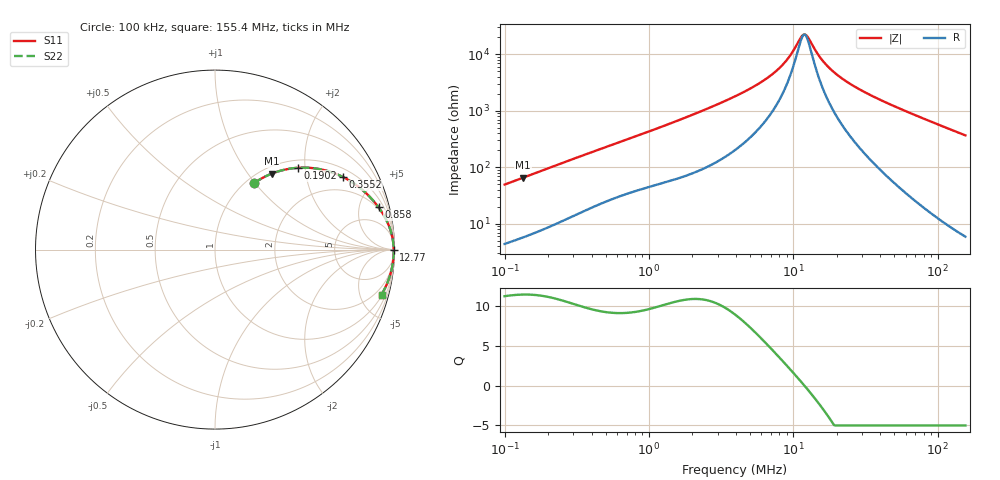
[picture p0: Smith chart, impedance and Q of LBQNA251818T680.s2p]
! LBQNA251818T680  S-PARAMETER MODEL  ( General Type )
! Model Generated by TAIYO YUDEN Corporation (http://www.ty-top.com)
! Version 1.0
! TAIYO YUDEN Control No. 191025NI43SB-FBB
! Copyright(c) 2019 TAIYO YUDEN CO.,LTD. All Rights Reserved.
! Product Description (link to TY-COMPAS)
! https://ds.yuden.co.jp/TYCOMPAS/or/detail?pn=LBQNA251818T680K&u=M
! Products Name : Inductors
! Characteristics :
!  Inductance : 68 uH , SRF(min) : 9.5 MHz , DC Resistance(max) : 1.95 Ohm
!  Rated Current : Saturation :70 mA , Temp Rise : 210 mA (20 degC)
!  Case Size : 2.5 x 1.8 / 0.098 x 0.071 [mm/inch] , Thickness : 1.8 / 0.071 [mm/inch]
!  (Conditions: Temperature = 25 degC , DC Bias Current/Voltage = 0A / 0V)
! External Node Assignments :
!  1  o---GGG---o  2
! GND o---------o GND
! Frequency Range : 0.1MHz  -  155.401204MHz  [ 402 STEP ]
# MHz S RI R 50
! Freq[MHz].  S11 Real  S11 Imag  S21 Real  S21 Imag  S12 Real  S12 Imag  S22 Real  S22 Imag
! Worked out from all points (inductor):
!   401 points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, 100 kHz to 155.4 MHz, reference 50 ohm
!   read as one part in series: L = 77.7 uH near 103.7 kHz
!   highest Q = 11.4 at 134.2 kHz (marker M1), where L = 77.6 uH
!   self-resonance near 11.87 MHz
!   S11 on the Smith chart (normalised r, x): 100 kHz: 1.09, +0.99; 190.2 kHz: 1.16, +1.83; 355.2 kHz: 1.34, +3.30; 858 kHz: 1.80, +7.44; 12.77 MHz: open; 155.4 MHz: 1.12, -7.36
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0.1  0.2168 0.3698  0.7832 -0.3698  0.7832 -0.3698  0.2168 0.3698
0.134171  0.3158 0.4231  0.6842 -0.4231  0.6842 -0.4231  0.3158 0.4231
0.190218  0.4605 0.4558  0.5395 -0.4558  0.5395 -0.4558  0.4605 0.4558
0.342427  0.7014 0.4099  0.2986 -0.4099  0.2986 -0.4099  0.7014 0.4099
0.355243  0.7141 0.4038  0.2859 -0.4038  0.2859 -0.4038  0.7141 0.4038
0.542044  0.832 0.3231  0.168 -0.3231  0.168 -0.3231  0.832 0.3231
0.858026  0.9115 0.2354  0.0885 -0.2354  0.0885 -0.2354  0.9115 0.2354
1.172566  0.9449 0.1834  0.0551 -0.1834  0.0551 -0.1834  0.9449 0.1834
3.942096  0.9909 0.0541  0.00909 -0.0541  0.00909 -0.0541  0.9909 0.0541
5.798004  0.9938 0.0318  0.00619 -0.0318  0.00619 -0.0318  0.9938 0.0318
7.637621  0.9949 0.0187  0.00515 -0.0187  0.00515 -0.0187  0.9949 0.0187
9.177924  0.9953 0.0107  0.00473 -0.0107  0.00473 -0.0107  0.9953 0.0107
11.65378  0.9956 0.000912  0.00442 -0.000912  0.00442 -0.000912  0.9956 0.000912
12.08994  0.9956 -0.000586  0.0044 0.000586  0.0044 0.000586  0.9956 -0.000586
12.77497  0.9956 -0.00284  0.00436 0.00284  0.00436 0.00284  0.9956 -0.00284
13.49882  0.9957 -0.0051  0.00434 0.0051  0.00434 0.0051  0.9957 -0.0051
16.22117  0.9956 -0.0128  0.00436 0.0128  0.00436 0.0128  0.9956 -0.0128
20.59702  0.9954 -0.0236  0.00459 0.0236  0.00459 0.0236  0.9954 -0.0236
28.66948  0.9945 -0.0409  0.0055 0.0409  0.0055 0.0409  0.9945 -0.0409
46.22367  0.9908 -0.0745  0.00921 0.0745  0.00921 0.0745  0.9908 -0.0745
86.32529  0.975 -0.1444  0.025 0.1444  0.025 0.1444  0.975 -0.1444
155.4012  0.9278 -0.2509  0.0722 0.2509  0.0722 0.2509  0.9278 -0.2509
